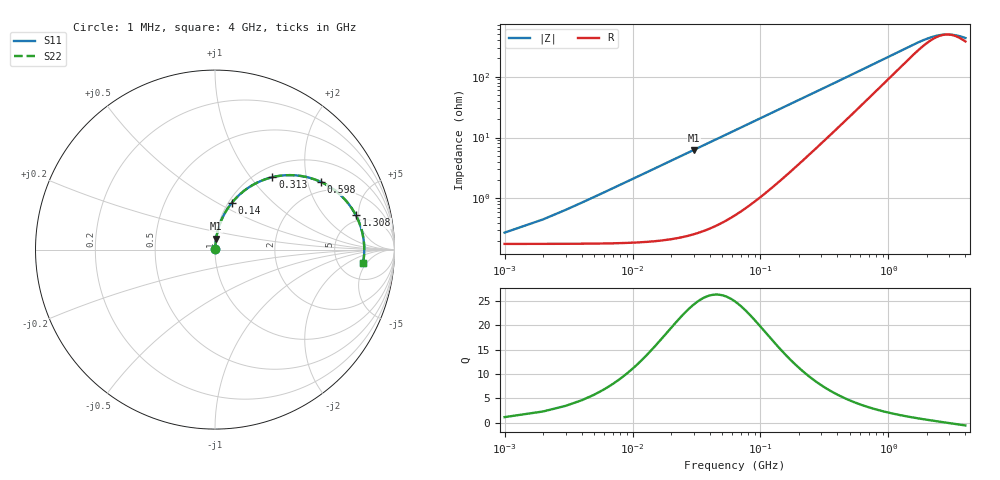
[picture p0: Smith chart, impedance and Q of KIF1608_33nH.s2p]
# MHz S RI R 50
!Freq ReS11 ImS11 ReS21 ImS21 ReS12 ImS12 ReS22 ImS22
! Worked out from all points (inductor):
!   4000 points, 1 MHz to 4 GHz, reference 50 ohm
!   read as one part in series: L = 33 nH near 21 MHz
!   highest Q = 24 at 30 MHz (marker M1), where L = 33 nH
!   self-resonance near 2.885 GHz
!   S11 on the Smith chart (normalised r, x): 1 MHz: 1.00, +0.00; 140 MHz: 1.04, +0.58; 313 MHz: 1.18, +1.29; 598 MHz: 1.64, +2.42; 1.308 GHz: 4.19, +4.62; 4 GHz: 8.59, -4.18
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1  0.00178 0.00206  0.9982 -0.00206  0.9982 -0.00206  0.00178 0.00206
11  0.0024 0.0227  0.9976 -0.0227  0.9976 -0.0227  0.0024 0.0227
23  0.00449 0.0473  0.9955 -0.0473  0.9955 -0.0473  0.00449 0.0473
30  0.00638 0.0616  0.9936 -0.0616  0.9936 -0.0616  0.00638 0.0616
37  0.00875 0.0758  0.9912 -0.0758  0.9912 -0.0758  0.00875 0.0758
46  0.0125 0.0938  0.9875 -0.0938  0.9875 -0.0938  0.0125 0.0938
70  0.0262 0.1404  0.9738 -0.1404  0.9738 -0.1404  0.0262 0.1404
101  0.0512 0.1964  0.9488 -0.1964  0.9488 -0.1964  0.0512 0.1964
140  0.0919 0.2583  0.9081 -0.2583  0.9081 -0.2583  0.0919 0.2583
215  0.188 0.3462  0.812 -0.3462  0.812 -0.3462  0.188 0.3462
313  0.3197 0.4034  0.6803 -0.4034  0.6803 -0.4034  0.3197 0.4034
452  0.4753 0.4108  0.5247 -0.4108  0.5247 -0.4108  0.4753 0.4108
598  0.5888 0.3776  0.4112 -0.3776  0.4112 -0.3776  0.5888 0.3776
668  0.6284 0.3568  0.3716 -0.3568  0.3716 -0.3568  0.6284 0.3568
937  0.7251 0.2775  0.2749 -0.2775  0.2749 -0.2775  0.7251 0.2775
1308  0.785 0.1912  0.215 -0.1912  0.215 -0.1912  0.785 0.1912
1334  0.7875 0.1861  0.2125 -0.1861  0.2125 -0.1861  0.7875 0.1861
1666  0.8107 0.1301  0.1893 -0.1301  0.1893 -0.1301  0.8107 0.1301
2001  0.8227 0.0856  0.1773 -0.0856  0.1773 -0.0856  0.8227 0.0856
2667  0.8313 0.0182  0.1687 -0.0182  0.1687 -0.0182  0.8313 0.0182
3334  0.8304 -0.0335  0.1696 0.0335  0.1696 0.0335  0.8304 -0.0335
4000  0.8247 -0.0763  0.1753 0.0763  0.1753 0.0763  0.8247 -0.0763
